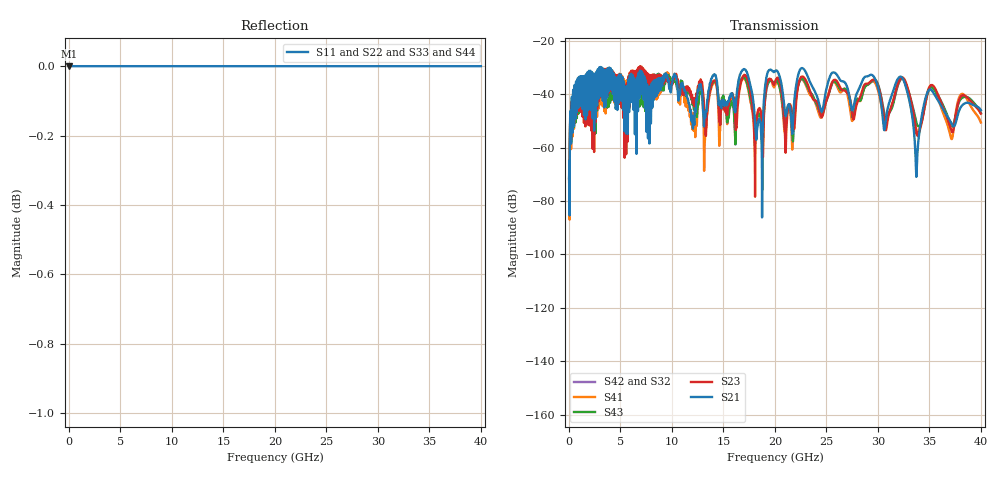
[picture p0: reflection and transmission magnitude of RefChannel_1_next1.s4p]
# GHz S RI R 50
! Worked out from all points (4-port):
!   4000 points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, 10 MHz to 40 GHz, reference 50 ohm
!   strongest paths, dB at 10 MHz, 10.01 GHz, 20.01 GHz, 30.01 GHz, 40 GHz:
!     S21: -71.3, -35.9, -31.5, -37.5, -46.0
!     S23: -71.5, -36.0, -35.6, -36.9, -47.3
!     S43: -71.9, -35.3, -35.5, -36.4, -47.1
!     S41: -72.9, -35.5, -36.7, -38.6, -50.6
!     S42: -, -, -, -, -
!     S32: -, -, -, -, -
!   lowest |S11| = 0.0 dB at 10 MHz (marker M1)
!   |S11| at or under -10 dB: nowhere
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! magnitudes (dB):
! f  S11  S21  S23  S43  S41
! 10 MHz  0.0  -71.3  -71.5  -71.9  -72.9
! 3.08 GHz  0.0  -30.1  -30.5  -31.1  -31.6
! 18.64 GHz  0.0  -53.3  -46.6  -50.4  -48.6
! 32.22 GHz  0.0  -33.5  -34.0  -34.4  -34.4
! 33.75 GHz  0.0  -70.2  -54.3  -50.9  -55.0
! 34.99 GHz  0.0  -38.3  -37.5  -38.1  -37.4
! 40 GHz  0.0  -46.0  -47.3  -47.1  -50.6
